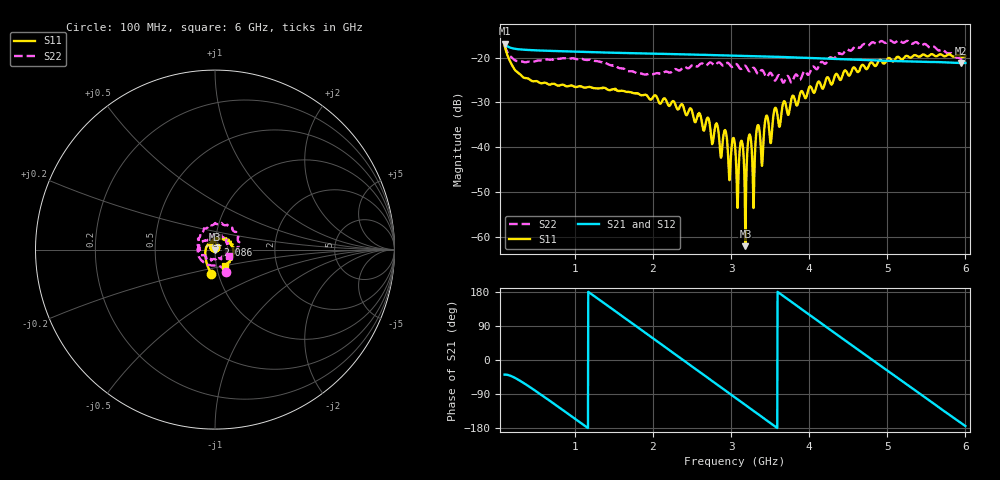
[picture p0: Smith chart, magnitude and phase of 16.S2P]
!Agilent Technologies,E5071C,MY46316741,A.11.02
!Date: Thu Dec 16 09:41:54 2021
!Data & Calibration Information:
!Freq	S11:SOLT4(ON)	S21:SOLT4(ON)	S12:SOLT4(ON)	S22:SOLT4(ON)
!PortZ  Port1:50+j0  Port2:50+j0
!Above PortZ is port z conversion or system Z0 setting when saving the data.
!When reading, reference impedance value at option line is always used.
# Hz S dB R 50
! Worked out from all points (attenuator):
!   1593 points, 100 MHz to 6 GHz, reference 50 ohm
!   highest |S21| = -16.90 dB at 100 MHz (marker M1); lowest = -21.2 dB at 5.941 GHz (marker M2)
!   lowest |S11| = -62.1 dB at 3.183 GHz (marker M3), VSWR 1.00, Z = 49.9 - j0.059 ohm
!   |S11| at or under -10 dB: start of sweep to end of sweep
!   |S22| runs from -25.6 to -16.2 dB; largest |S21 - S12| = 0.0006
!   S11 on the Smith chart (normalised r, x): 100 MHz: 0.93, -0.25; 2.086 GHz: 1.03, +0.06; 6 GHz: 1.09, -0.20
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1e8  -17.33 -98.7  -16.90 -38.6  -16.91 -38.5  -17.22 -64.0
3.44598e8  -24.46 -154.2  -18.24 -60.8  -18.24 -60.8  -21.01 -88.5
1.085804e9  -26.44 137.2  -18.72 -167.5  -18.72 -167.5  -20.26 -179.6
2.067902e9  -29.63 69.5  -19.15 47.2  -19.15 47.2  -23.45 124.6
2.086432e9  -30.26 63.8  -19.15 44.4  -19.16 44.5  -23.59 123.9
2.701633e9  -33.38 1.6  -19.41 -47.1  -19.42 -47.0  -21.46 79.0
2.979585e9  -47.33 -47.3  -19.53 -88.5  -19.54 -88.4  -21.50 53.5
3.05e9  -39.65 -38.8  -19.57 -98.9  -19.58 -98.8  -21.53 40.1
3.083354e9  -53.52 -88.3  -19.58 -103.9  -19.59 -103.8  -21.67 40.4
3.135239e9  -38.57 -92.2  -19.61 -111.7  -19.62 -111.5  -22.46 28.8
3.183417e9  -62.06 -131.6  -19.63 -118.8  -19.64 -118.7  -21.83 25.4
3.235302e9  -37.17 -138.4  -19.66 -126.6  -19.66 -126.4  -23.07 16.7
3.287186e9  -53.56 -150.3  -19.68 -134.2  -19.69 -134.1  -22.27 8.8
3.342776e9  -35.07 -170.0  -19.70 -142.5  -19.71 -142.3  -23.61 -0.3
3.394661e9  -44.14 -172.4  -19.72 -150.2  -19.73 -150.0  -22.77 -11.3
3.453957e9  -32.94 171.4  -19.75 -159.1  -19.75 -158.9  -24.34 -23.0
3.505842e9  -39.07 168.3  -19.77 -166.8  -19.78 -166.7  -23.39 -33.1
3.565138e9  -31.20 156.1  -19.81 -175.7  -19.81 -175.6  -25.11 -47.7
4.035804e9  -27.04 118.3  -20.11 114.4  -20.11 114.5  -22.23 -156.2
5.017902e9  -20.09 26.0  -20.73 -30.4  -20.73 -30.2  -16.28 64.1
5.940704e9  -19.76 -52.6  -21.20 -165.8  -21.19 -165.4  -20.30 -19.2
6e9  -19.62 -59.5  -21.19 -174.3  -21.18 -174.1  -21.12 -23.6
